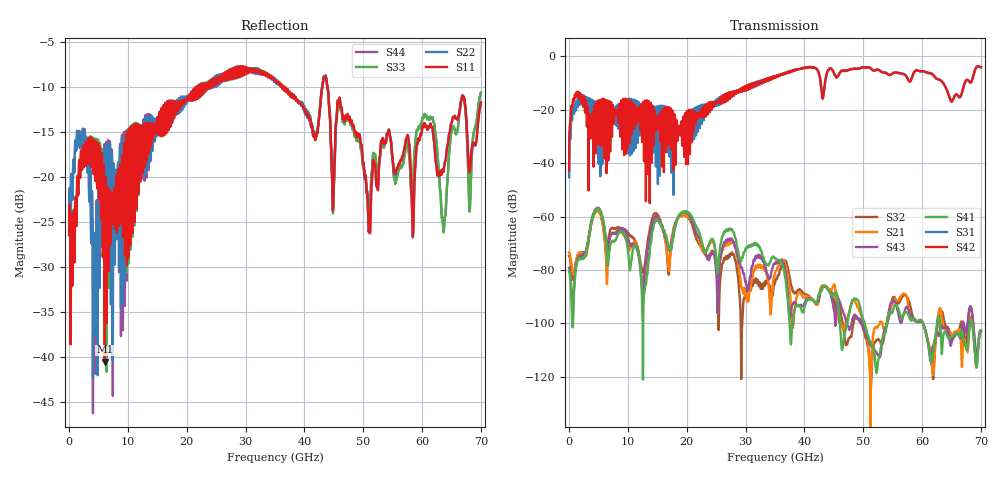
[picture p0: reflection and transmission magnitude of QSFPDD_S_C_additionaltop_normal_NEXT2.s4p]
! AWR Design Environment (8415) Thu Dec 20 13:41:51 2018
! Document = 'CHANNEL TEST'
! nPorts: 4, nXvals: 7001
# HZ S DB R 50
!Freq DBS11 AngS11 DBS12 AngS12 DBS13 AngS13 DBS14 AngS14
!	DBS21 AngS21 DBS22 AngS22 DBS23 AngS23 DBS24 AngS24
!	DBS31 AngS31 DBS32 AngS32 DBS33 AngS33 DBS34 AngS34
!	DBS41 AngS41 DBS42 AngS42 DBS43 AngS43 DBS44 AngS44
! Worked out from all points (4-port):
!   7000 points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, 10 MHz to 70 GHz, reference 50 ohm
!   strongest paths, dB at 10 MHz, 17.51 GHz, 35.01 GHz, 52.51 GHz, 70 GHz:
!     S42: -42.7, -23.6, -7.5, -5.0, -4.0
!     S31: -45.3, -23.9, -7.5, -5.0, -4.0
!     S41: -80.5, -69.9, -75.5, -114.3, -102.6
!     S43: -79.1, -69.4, -77.6, -111.6, -103.0
!     S21: -73.4, -68.5, -81.2, -101.1, -102.6
!     S32: -74.7, -67.1, -84.6, -105.8, -103.0
!   lowest |S11| = -40.5 dB at 6.06 GHz (marker M1), VSWR 1.02, Z = 49.4 + j0.738 ohm
!   |S11| at or under -10 dB: start of sweep to 21.77 GHz; 36.5 GHz to 43.04 GHz (6.538 GHz wide, 16.4 % of centre); 43.94 GHz to end of sweep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
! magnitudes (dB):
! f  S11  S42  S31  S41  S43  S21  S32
! 10 MHz  -26.5  -42.7  -45.3  -80.5  -79.1  -73.4  -74.7
! 1.29 GHz  -23.5  -13.2  -16.8  -78.1  -77.3  -75.8  -75.9
! 4.62 GHz  -16.1  -17.0  -20.6  -57.5  -57.1  -58.2  -57.8
! 6.06 GHz  -40.5  -29.1  -18.8  -64.6  -65.0  -67.8  -68.8
! 30.8 GHz  -8.1  -11.1  -11.4  -70.9  -82.7  -87.1  -87.3
! 63.65 GHz  -19.4  -10.2  -10.2  -104.0  -101.6  -101.9  -97.8
! 70 GHz  -11.8  -4.0  -4.0  -102.6  -103.0  -102.6  -103.0
